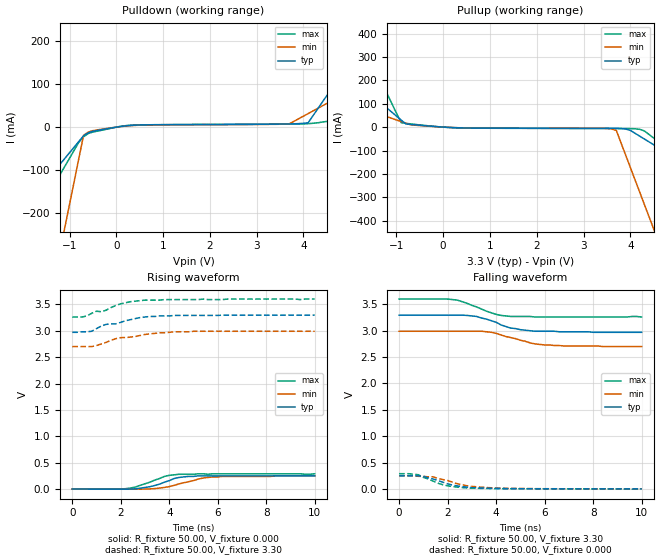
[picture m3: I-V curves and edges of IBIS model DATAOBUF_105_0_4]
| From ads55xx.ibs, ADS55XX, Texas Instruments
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|   Model DATAOBUF_105_0_4
[Model]   DATAOBUF_105_0_4
Model_type   Output
Polarity   Non-Inverting
Vmeas =   1.65V
C_comp   3.00pF   3.00pF   3.00pF
[Temperature Range]   50.00   0.10k   -20.00
[Voltage Range]   3.30V   3.00V   3.60V
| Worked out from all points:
|   slope of the pulldown table from 0 to 0.495 V, typ, clamps not added: 98.6 ohm
|   slope of the pullup table from 0 to 0.495 V, typ, clamps not added: 123 ohm
|   rising waveform, R_fixture 50.00, V_fixture 0.000: 20-80 % time 953ps typ, 1.27ns min, 1.04ns max; typ from 0 V to 0.25 V
|   rising waveform, R_fixture 50.00, V_fixture 3.30: 20-80 % time 1.62ns typ, 1.79ns min, 1.43ns max; typ from 2.97 V to 3.29 V
|   falling waveform, R_fixture 50.00, V_fixture 3.30: 20-80 % time 1.35ns typ, 1.4ns min, 1.16ns max; typ from 3.29 V to 2.97 V
|   falling waveform, R_fixture 50.00, V_fixture 0.000: 20-80 % time 1.22ns typ, 1.36ns min, 1.07ns max; typ from 0.25 V to 0.002 V
[Pulldown]
| voltage   I(typ)   I(min)   I(max)
-3.3V     -362.7mA   -1.413A    -504mA
-2.3V     -230.9mA   -877mA     -316.4mA
-1.9V     -178.2mA   -662.5mA   -241.3mA
-1.5V     -125.5mA   -448mA     -166.3mA
-1V       -59.57mA   -179.9mA   -72.47mA
-700mV    -20.03mA   -19.07mA   -22.51mA
-500mV    -9.68mA    -8.16mA    -11.47mA
400mV     4.6mA      4.04mA     4.95mA
3.7V      7.39mA     7.83mA     7.1mA
4.1V      10.18mA    31.55mA    8.06mA
5.5V      232.2mA    114.6mA    29.88mA
6.6V      406.7mA    179.8mA    48.03mA
[Pullup]
| voltage   I(typ)   I(min)   I(max)
-3.3V     433.9mA    190.1mA    1.012A
-1.9V     198.7mA    93.13mA    433mA
-900mV    30.71mA    23.83mA    19.13mA
-800mV    13.91mA    16.9mA     16.35mA
300mV     -2.6mA     -2.4mA     -3.32mA
3.6V      -5.21mA    -7.64mA    -5.87mA
3.7V      -5.32mA    -14.21mA   -5.9mA
4V        -13.87mA   -172.3mA   -6.24mA
4.2V      -38.47mA   -277.8mA   -9.33mA
4.3V      -50.77mA   -330.5mA   -16.27mA
4.5V      -75.37mA   -435.9mA   -46.65mA
6.6V      -333.7mA   -1.543A    -365.6mA
[Ramp]
| variable   typ   min   max
dV/dt_r   0.15/1.03n   0.15/1.25n   0.17/0.98n
dV/dt_f   0.19/1.28n   0.18/1.41n   0.20/1.10n
R_load = 50.00
[Rising Waveform]
R_fixture = 50.00
V_fixture = 0.000
V_fixture_min = 0.000
V_fixture_max = 0.000
| time   V(typ)   V(min)   V(max)
0s        18.56nV    22.43nV    39.39nV
1.8ns     -1.47mV    -650uV     -1.11mV
2.4ns     54.12uV    -1.61mV    19.79mV
3.2ns     44.75mV    3.09mV     130mV
3.8ns     130mV      31mV       240mV
4.2ns     200mV      70.09mV    270mV
4.4ns     220mV      97.65mV    280mV
5.4ns     250mV      210mV      290mV
5.8ns     250mV      230mV      290mV
10ns      250mV      250mV      290mV
[Rising Waveform]
R_fixture = 50.00
V_fixture = 3.30
V_fixture_min = 3.00
V_fixture_max = 3.60
| time   V(typ)   V(min)   V(max)
0s        2.97V      2.7V       3.26V
400ps     2.98V      2.7V       3.26V
800ps     2.99V      2.7V       3.33V
1ns       3.04V      2.72V      3.37V
1.2ns     3.09V      2.75V      3.36V
1.4ns     3.12V      2.78V      3.39V
2ns       3.16V      2.87V      3.51V
3ns       3.26V      2.93V      3.58V
5ns       3.29V      2.99V      3.59V
10ns      3.295V     2.99V      3.6V
[Falling Waveform]
R_fixture = 50.00
V_fixture = 3.30
V_fixture_min = 3.00
V_fixture_max = 3.60
| time   V(typ)   V(min)   V(max)
0s        3.295V     2.99V      3.6V
2ns       3.295V     2.99V      3.6V
2.4ns     3.295V     2.99V      3.58V
3.2ns     3.27V      2.99V      3.45V
4ns       3.16V      2.95V      3.31V
4.6ns     3.05V      2.87V      3.27V
5.4ns     3V         2.77V      3.27V
6ns       2.99V      2.73V      3.26V
6.8ns     2.98V      2.71V      3.26V
10ns      2.97V      2.7V       3.26V
[Falling Waveform]
R_fixture = 50.00
V_fixture = 0.000
V_fixture_min = 0.000
V_fixture_max = 0.000
| time   V(typ)   V(min)   V(max)
0s        250mV      250mV      290mV
800ps     250mV      240mV      270mV
1ns       240mV      240mV      220mV
1.4ns     190mV      230mV      150mV
1.6ns     160mV      200mV      110mV
2ns       97.47mV    160mV      60.72mV
2.4ns     58.23mV    100mV      36.32mV
2.8ns     35.08mV    61.06mV    19.99mV
4.4ns     7.88mV     12.97mV    5.4mV
10ns      1.71mV     2.06mV     1.39mV
